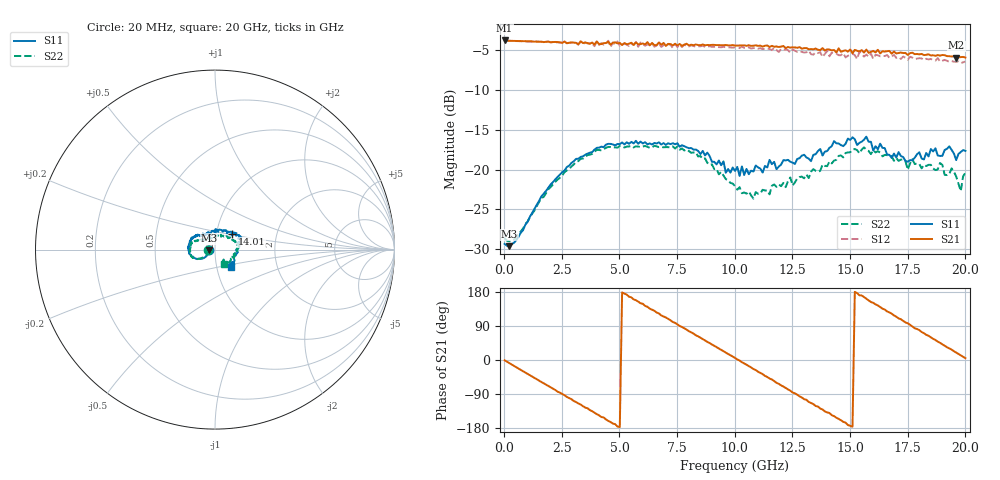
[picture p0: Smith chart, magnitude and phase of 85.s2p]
!Agilent Technologies,N5230A,US43500223,A.07.50.48
!Agilent N5230A: A.07.50.48
!Date: Thursday, October 08, 2015 16:12:28
!Correction: S11(Full 2 Port(1,2))
!S21(Full 2 Port(1,2))
!S12(Full 2 Port(1,2))
!S22(Full 2 Port(1,2))
!S2P File: Measurements: S11, S21, S12, S22:
# Hz S  RI  R 50
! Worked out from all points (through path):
!   201 points, 20 MHz to 20 GHz, reference 50 ohm
!   highest |S21| = -3.78 dB at 20 MHz (marker M1); lowest = -5.9 dB at 19.6 GHz (marker M2)
!   group delay of S21, straight-line fit = 99.1 ps
!   lowest |S11| = -29.6 dB at 219.8 MHz (marker M3), VSWR 1.07, Z = 46.8 - j0.408 ohm
!   |S11| at or under -10 dB: start of sweep to end of sweep
!   |S22| runs from -29.0 to -17.0 dB; largest |S21 - S12| = 0.076
!   S11 on the Smith chart (normalised r, x): 20 MHz: 0.93, +0.00; 14.01 GHz: 1.19, +0.21; 20 GHz: 1.18, -0.23
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2e7  -0.0341 0.000389  0.6469 -0.00858  0.646 -0.00966  -0.0371 -0.000389
2.198e8  -0.0327 -0.00436  0.6375 -0.0904  0.637 -0.0913  -0.0353 -0.00361
1.8182e9  -0.0585 -0.0446  0.2665 -0.5758  0.256 -0.5795  -0.0595 -0.039
2.6174e9  -0.0848 -0.0504  -0.0331 -0.637  -0.042 -0.6274  -0.0822 -0.0502
3.4166e9  -0.1108 -0.0488  -0.328 -0.5296  -0.3449 -0.5107  -0.1062 -0.0495
4.9151e9  -0.1443 -0.0123  -0.6185 -0.0482  -0.6378 -0.0238  -0.1354 -0.023
5.7143e9  -0.1511 0.0119  -0.5831 0.2369  -0.579 0.2541  -0.14 -0.00294
6.7133e9  -0.1406 0.0469  -0.3401 0.5287  -0.3163 0.5325  -0.1368 0.0207
8.3117e9  -0.1059 0.0816  0.2566 0.5539  0.2747 0.5231  -0.1207 0.0435
1.001e10  -0.0433 0.088  0.5981 0.0559  0.5854 0.0234  -0.0555 0.056
1.08092e10  -0.0205 0.0951  0.5483 -0.241  0.5178 -0.2597  -0.0181 0.0632
1.17083e10  0.0164 0.1106  0.334 -0.487  0.3037 -0.4961  0.0139 0.0794
1.25075e10  0.0404 0.103  0.0424 -0.5847  0.0217 -0.5683  0.0343 0.0717
1.34066e10  0.0718 0.1007  -0.2523 -0.5099  -0.2595 -0.4586  0.0677 0.0745
1.4006e10  0.097 0.0876  -0.4254 -0.3787  -0.439 -0.3408  0.0896 0.0549
1.54046e10  0.1332 0.0628  -0.5452 0.0877  -0.5432 0.0845  0.1239 0.0252
1.67033e10  0.1236 0.00649  -0.3235 0.4523  -0.2711 0.4241  0.123 -0.00628
1.81019e10  0.0952 -0.0687  0.1476 0.5118  0.162 0.4719  0.0883 -0.0508
1.93007e10  0.0987 -0.0991  0.4442 0.261  0.4202 0.2226  0.0592 -0.0726
1.96004e10  0.0833 -0.0788  0.4753 0.17  0.4542 0.1385  0.0449 -0.0787
1.98002e10  0.1032 -0.0775  0.497 0.1087  0.4612 0.0667  0.0479 -0.0553
2e10  0.0905 -0.0949  0.5037 0.0422  0.4766 0.00923  0.0492 -0.0821
